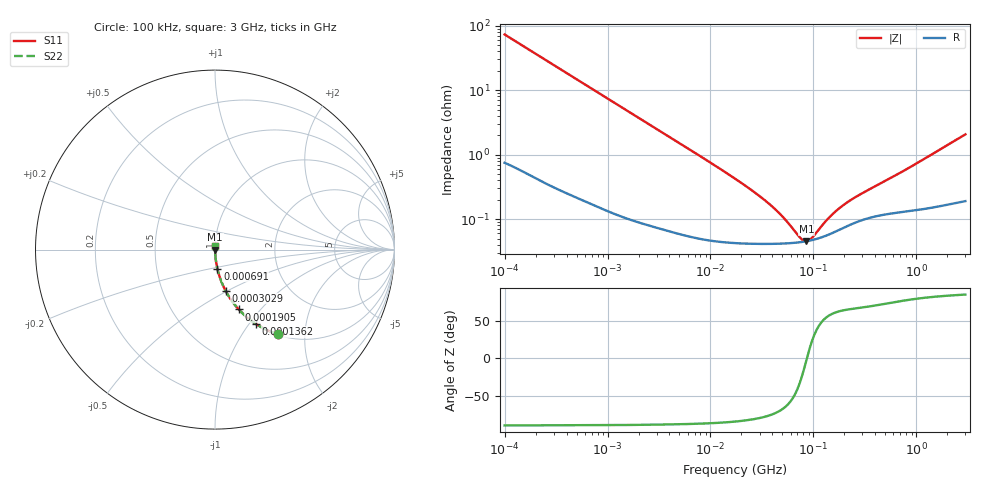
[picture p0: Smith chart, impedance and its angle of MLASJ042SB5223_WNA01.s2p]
! MLASJ042SB5223_WNA01  S-PARAMETER MODEL  ( Standard Model )
! Model Generated by TAIYO YUDEN Corporation (http://www.ty-top.com)
! Version 1.0
! TAIYO YUDEN Control No. 220601
! Copyright(c) 2010 TAIYO YUDEN CO.,LTD. All Rights Reserved.
! Product Description (link to TY-COMPAS)
! https://ds.yuden.co.jp/TYCOMPAS/or/detail?pn=MLASJ042SB5223KWNA01&u=M
! Products Name : Multilayer Ceramic Capacitors
! Characteristics :
!  Capacitance : 0.022 [uF] , Rated Voltage : 6.3 [V] , TCC : X5R
!  Case Size : 0.4 x 0.2 / 0.016 x 0.008 [mm/inch] , Thickness : 0.2 / 0.008 [mm/inch]
!  (Conditions: Temperature = 25 [degC] , DC Bias Voltage = 0 [V])
! External Node Assignments :
!  1  o---| |---o  2
! GND o---------o GND
! Frequency Range : 100kHz  -  3GHz  [ 401 STEP ]
# MHZ S RI R 50
! Freq[MHz].  S11 Real  S11 Imag  S21 Real  S21 Imag  S12 Real  S12 Imag  S22 Real  S22 Imag
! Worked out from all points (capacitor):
!   401 points, 100 kHz to 3 GHz, reference 50 ohm
!   read as one part in series: C = 21.7 nF near 105.3 kHz
!   lowest |Z| = 45.4 mohm at 85.61 MHz (marker M1)
!   series resonance near 86.57 MHz, so ESL is about 160 pH
!   S11 on the Smith chart (normalised r, x): 100 kHz: 1.01, -1.46; 136.2 kHz: 1.01, -1.08; 190.5 kHz: 1.01, -0.77; 302.9 kHz: 1.01, -0.49; 691 kHz: 1.00, -0.21; 3 GHz: 1.00, +0.04
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0.1  0.3504 -0.472  0.6496 0.472  0.6496 0.472  0.3504 -0.472
0.136243  0.2274 -0.4137  0.7726 0.4137  0.7726 0.4137  0.2274 -0.4137
0.190467  0.1327 -0.3335  0.8673 0.3335  0.8673 0.3335  0.1327 -0.3335
0.302894  0.0586 -0.2287  0.9414 0.2287  0.9414 0.2287  0.0586 -0.2287
0.562235  0.019 -0.1291  0.981 0.1291  0.981 0.1291  0.019 -0.1291
0.690972  0.0131 -0.1059  0.9869 0.1059  0.9869 0.1059  0.0131 -0.1059
1.350433  0.00414 -0.055  0.9959 0.055  0.9959 0.055  0.00414 -0.055
3.161081  0.00128 -0.0237  0.9987 0.0237  0.9987 0.0237  0.00128 -0.0237
17.7727  0.00044 -0.00411  0.9996 0.00411  0.9996 0.00411  0.00044 -0.00411
27.54426  0.000419 -0.00249  0.9996 0.00249  0.9996 0.00249  0.000419 -0.00249
38.50681  0.000415 -0.00159  0.9996 0.00159  0.9996 0.00159  0.000415 -0.00159
51.12795  0.000419 -0.000973  0.9996 0.000973  0.9996 0.000973  0.000419 -0.000973
75.25761  0.000439 -0.000248  0.9996 0.000248  0.9996 0.000248  0.000439 -0.000248
81.30716  0.000447 -0.00011  0.9996 0.00011  0.9996 0.00011  0.000447 -0.00011
85.60801  0.000454 -1.95e-05  0.9995 1.95e-05  0.9995 1.95e-05  0.000454 -1.95e-05
90.13636  0.000461 7.12e-05  0.9995 -7.12e-05  0.9995 -7.12e-05  0.000461 7.12e-05
97.38194  0.000473 0.000207  0.9995 -0.000207  0.9995 -0.000207  0.000473 0.000207
139.694  0.000572 0.000852  0.9994 -0.000852  0.9994 -0.000852  0.000572 0.000852
190.323  0.000717 0.00143  0.9993 -0.00143  0.9993 -0.00143  0.000717 0.00143
273.0175  0.000922 0.00213  0.9991 -0.00213  0.9991 -0.00213  0.000922 0.00213
547.5153  0.00122 0.00404  0.9988 -0.00404  0.9988 -0.00404  0.00122 0.00404
3000  0.00232 0.0205  0.9977 -0.0205  0.9977 -0.0205  0.00232 0.0205
